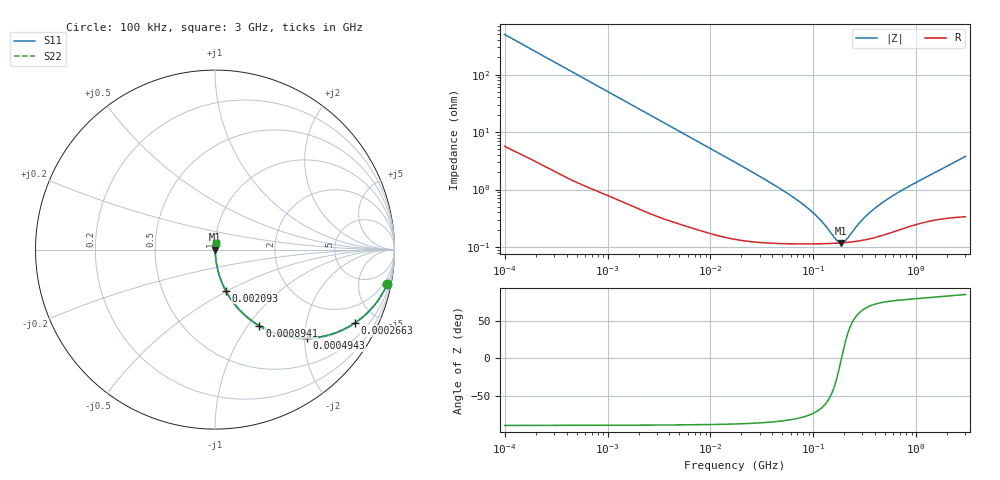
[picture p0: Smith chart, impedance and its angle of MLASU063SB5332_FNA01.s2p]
! MLASU063SB5332_FNA01  S-PARAMETER MODEL  ( Standard Model )
! Model Generated by TAIYO YUDEN Corporation (http://www.ty-top.com)
! Version 1.0
! TAIYO YUDEN Control No. 220601
! Copyright(c) 2013 TAIYO YUDEN CO.,LTD. All Rights Reserved.
! Product Description (link to TY-COMPAS)
! https://ds.yuden.co.jp/TYCOMPAS/or/detail?pn=MLASU063SB5332KFNA01&u=M
! Products Name : Multilayer Ceramic Capacitors
! Characteristics :
!  Capacitance : 3300 [pF] , Rated Voltage : 50 [V] , TCC : B / X5R
!  Case Size : 0.6 x 0.3 / 0.024 x 0.012 [mm/inch] , Thickness : 0.3 / 0.012 [mm/inch]
!  (Conditions: Temperature = 25 [degC] , DC Bias Voltage = 0 [V])
! External Node Assignments :
!  1  o---| |---o  2
! GND o---------o GND
! Frequency Range : 100kHz  -  3GHz  [ 401 STEP ]
# MHZ S RI R 50
! Freq[MHz].  S11 Real  S11 Imag  S21 Real  S21 Imag  S12 Real  S12 Imag  S22 Real  S22 Imag
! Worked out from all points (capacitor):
!   401 points, 100 kHz to 3 GHz, reference 50 ohm
!   read as one part in series: C = 3.18 nF near 105.3 kHz
!   lowest |Z| = 118 mohm at 185.5 MHz (marker M1)
!   series resonance near 187.5 MHz, so ESL is about 230 pH
!   S11 on the Smith chart (normalised r, x): 100 kHz: 1, -10; 266.3 kHz: 1.05, -3.78; 494.3 kHz: 1.03, -2.05; 894.1 kHz: 1.02, -1.14; 2.093 MHz: 1.01, -0.49; 3 GHz: 1.01, +0.08
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0.1  0.9595 -0.1915  0.0405 0.1915  0.0405 0.1915  0.9595 -0.1915
0.167439  0.8969 -0.2982  0.1031 0.2982  0.1031 0.2982  0.8969 -0.2982
0.266273  0.7785 -0.4091  0.2215 0.4091  0.2215 0.4091  0.7785 -0.4091
0.372249  0.6458 -0.472  0.3542 0.472  0.3542 0.472  0.6458 -0.472
0.494258  0.5112 -0.4933  0.4888 0.4933  0.4888 0.4933  0.5112 -0.4933
0.562235  0.4482 -0.4906  0.5518 0.4906  0.5518 0.4906  0.4482 -0.4906
0.894104  0.2473 -0.4239  0.7527 0.4239  0.7527 0.4239  0.2473 -0.4239
1.350433  0.1289 -0.3269  0.8711 0.3269  0.8711 0.3269  0.1289 -0.3269
2.092911  0.0602 -0.2289  0.9398 0.2289  0.9398 0.2289  0.0602 -0.2289
3.161081  0.0288 -0.1573  0.9712 0.1573  0.9712 0.1573  0.0288 -0.1573
6.674626  0.00805 -0.0767  0.992 0.0767  0.992 0.0767  0.00805 -0.0767
17.7727  0.00219 -0.029  0.9978 0.029  0.9978 0.029  0.00219 -0.029
52.46276  0.00123 -0.00918  0.9988 0.00918  0.9988 0.00918  0.00123 -0.00918
97.38194  0.00115 -0.00392  0.9989 0.00392  0.9989 0.00392  0.00115 -0.00392
122.8043  0.00115 -0.00243  0.9989 0.00243  0.9989 0.00243  0.00115 -0.00243
167.3121  0.00116 -0.000636  0.9988 0.000636  0.9988 0.000636  0.00116 -0.000636
185.4806  0.00118 -6.09e-05  0.9988 6.09e-05  0.9988 6.09e-05  0.00118 -6.09e-05
205.6221  0.0012 0.000513  0.9988 -0.000513  0.9988 -0.000513  0.0012 0.000513
280.1453  0.00128 0.00228  0.9987 -0.00228  0.9987 -0.00228  0.00128 0.00228
344.2911  0.00139 0.00355  0.9986 -0.00355  0.9986 -0.00355  0.00139 0.00355
547.5153  0.00178 0.00692  0.9982 -0.00692  0.9982 -0.00692  0.00178 0.00692
3000  0.00476 0.0373  0.9952 -0.0373  0.9952 -0.0373  0.00476 0.0373
